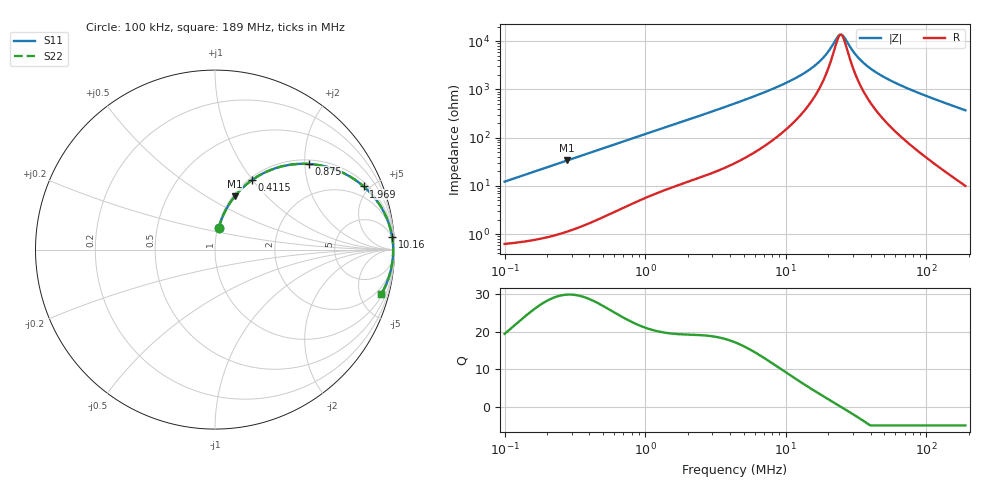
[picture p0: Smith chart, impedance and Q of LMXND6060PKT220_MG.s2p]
! LMXND6060PKT220_MG  S-PARAMETER MODEL  ( General Type )
! Model Generated by TAIYO YUDEN Corporation (http://www.ty-top.com)
! Version 1.0
! TAIYO YUDEN Control No. 191025NI43SB-FBB
! Copyright(c) 2019 TAIYO YUDEN CO.,LTD. All Rights Reserved.
! Product Description (link to TY-COMPAS)
! https://ds.yuden.co.jp/TYCOMPAS/or/detail?pn=LMXND6060PKT220MMG&u=M
! Products Name : Inductors
! Characteristics :
!  Inductance : 22 uH , SRF(min) : 16 MHz , DC Resistance(max) : 0.36 Ohm
!  Rated Current : Saturation :950 mA , Temp Rise : 1000 mA
!  Case Size : 6.0 x 6.0 / 0.236 x 0.236 [mm/inch] , Thickness : 1.4 / 0.055 [mm/inch]
!  (Conditions: Temperature = 25 degC , DC Bias Current/Voltage = 0A / 0V)
! External Node Assignments :
!  1  o---GGG---o  2
! GND o---------o GND
! Frequency Range : 0.1MHz  -  189.042664MHz  [ 402 STEP ]
# MHz S RI R 50
! Freq[MHz].  S11 Real  S11 Imag  S21 Real  S21 Imag  S12 Real  S12 Imag  S22 Real  S22 Imag
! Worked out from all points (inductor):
!   401 points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, 100 kHz to 189 MHz, reference 50 ohm
!   read as one part in series: L = 19.5 uH near 103.8 kHz
!   highest Q = 29.9 at 276.9 kHz (marker M1), where L = 19.4 uH
!   self-resonance near 24.19 MHz
!   S11 on the Smith chart (normalised r, x): 100 kHz: 1.01, +0.25; 411.5 kHz: 1.03, +1.00; 875 kHz: 1.10, +2.09; 1.969 MHz: 1.24, +4.60; 10.16 MHz: 4, +28; 189 MHz: 1.20, -7.38
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0.1  0.0208 0.1193  0.9792 -0.1193  0.9792 -0.1193  0.0208 0.1193
0.176093  0.051 0.2023  0.949 -0.2023  0.949 -0.2023  0.051 0.2023
0.276908  0.11 0.2966  0.89 -0.2966  0.89 -0.2966  0.11 0.2966
0.353854  0.1643 0.354  0.8357 -0.354  0.8357 -0.354  0.1643 0.354
0.411486  0.2077 0.3886  0.7923 -0.3886  0.7923 -0.3886  0.2077 0.3886
0.623111  0.3659 0.462  0.6341 -0.462  0.6341 -0.462  0.3659 0.462
0.875006  0.5216 0.4773  0.4784 -0.4773  0.4784 -0.4773  0.5216 0.4773
1.252125  0.6786 0.4428  0.3214 -0.4428  0.3214 -0.4428  0.6786 0.4428
1.968979  0.8288 0.3517  0.1712 -0.3517  0.1712 -0.3517  0.8288 0.3517
4.347904  0.9535 0.1836  0.0465 -0.1836  0.0465 -0.1836  0.9535 0.1836
10.15998  0.9871 0.0702  0.0129 -0.0702  0.0129 -0.0702  0.9871 0.0702
15.38522  0.9914 0.0342  0.00862 -0.0342  0.00862 -0.0342  0.9914 0.0342
18.5788  0.9923 0.0199  0.00773 -0.0199  0.00773 -0.0199  0.9923 0.0199
23.29778  0.9927 0.00373  0.00726 -0.00373  0.00726 -0.00373  0.9927 0.00373
24.65407  0.9928 -0.00026  0.00723 0.00026  0.00723 0.00026  0.9928 -0.00026
26.08933  0.9928 -0.00426  0.00723 0.00426  0.00723 0.00426  0.9928 -0.00426
30.3385  0.9926 -0.015  0.00741 0.015  0.00741 0.015  0.9926 -0.015
35.27973  0.9922 -0.0261  0.00785 0.0261  0.00785 0.0261  0.9922 -0.0261
42.60291  0.9912 -0.0408  0.00882 0.0408  0.00882 0.0408  0.9912 -0.0408
54.44117  0.989 -0.0621  0.011 0.0621  0.011 0.0621  0.989 -0.0621
92.31806  0.9778 -0.1214  0.0222 0.1214  0.0222 0.1214  0.9778 -0.1214
189.0427  0.9257 -0.249  0.0743 0.249  0.0743 0.249  0.9257 -0.249
